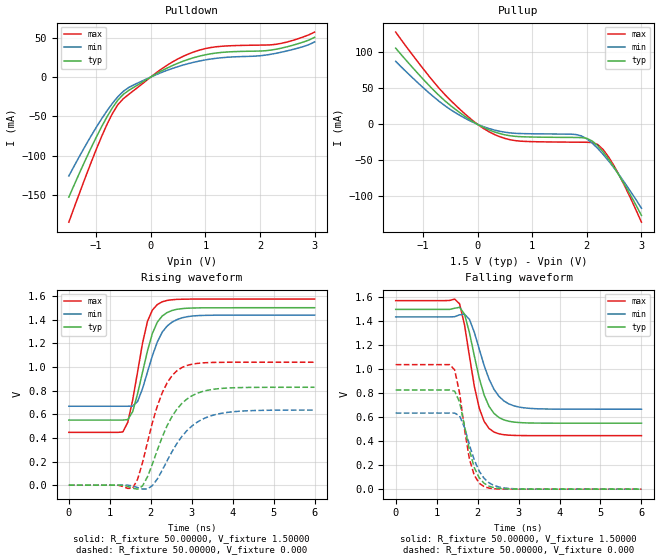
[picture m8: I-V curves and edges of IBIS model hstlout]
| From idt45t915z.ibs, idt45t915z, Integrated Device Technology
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|   Model hstlout
[Model]   hstlout
Model_type   Output
Polarity   Non-Inverting
Vmeas =  0.75000V
C_comp   5.00000pF   5.00000pF   5.00000pF
[Temperature Range]   45.00000   0.14000k   -30.00000
[Voltage Range]   1.50000V   1.40000V   1.60000V
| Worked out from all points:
|   slope of the pulldown table from 0 to 0.225 V, typ, clamps not added: 25.7 ohm
|   slope of the pullup table from 0 to 0.225 V, typ, clamps not added: 27.7 ohm
|   rising waveform, R_fixture 50.00000, V_fixture 1.50000: 20-80 % time 422ps typ, 461ps min, 368ps max; typ from 0.55 V to 1.5 V
|   rising waveform, R_fixture 50.00000, V_fixture 0.000: 20-80 % time 662ps typ, 754ps min, 540ps max; typ from 0 V to 0.828 V
|   falling waveform, R_fixture 50.00000, V_fixture 1.50000: 20-80 % time 419ps typ, 483ps min, 354ps max; typ from 1.5 V to 0.55 V
|   falling waveform, R_fixture 50.00000, V_fixture 0.000: 20-80 % time 340ps typ, 400ps min, 296ps max; typ from 0.828 V to 0 V
[Pulldown]
| voltage   I(typ)   I(min)   I(max)
-1.5V     -152.2mA   -125.4mA   -184mA
-1V       -76.61mA   -64mA      -92.15mA
-700mV    -38.83mA   -33.15mA   -46.03mA
-600mV    -29.09mA   -24.77mA   -34.85mA
-400mV    -16.8mA    -13.12mA   -21.77mA
100mV     4.071mA    3.04mA     5.393mA
500mV     17.6mA     13.29mA    23.07mA
900mV     26.67mA    20.45mA    34.32mA
1.3V      31.24mA    24.53mA    39.05mA
2.3V      35.32mA    30.19mA    41.59mA
2.7V      42.32mA    36.77mA    48.64mA
3V        50.37mA    44.55mA    57.01mA
[Pullup]
| voltage   I(typ)   I(min)   I(max)
-1.5V     106mA      87.68mA    128.3mA
-1V       63.03mA    51.23mA    77.62mA
-600mV    32.8mA     26mA       41.46mA
-100mV    4.501mA    3.42mA     5.936mA
200mV     -7.39mA    -5.559mA   -9.876mA
700mV     -16.74mA   -12.49mA   -22.72mA
1.8V      -18.22mA   -14.08mA   -24.77mA
2V        -19.46mA   -20.18mA   -24.89mA
2.2V      -29.78mA   -33.53mA   -28.11mA
2.3V      -38.45mA   -41.87mA   -35.18mA
2.5V      -59.91mA   -60.81mA   -57.87mA
3V        -126.6mA   -116.6mA   -136mA
[Ramp]
| variable   typ   min   max
dV/dt_r   0.49650/0.71046n   0.38094/0.80872n   0.62340/0.57985n
dV/dt_f   0.56976/0.43675n   0.47046/0.50537n   0.67140/0.37589n
R_load = 50.00000
[Rising Waveform]
R_fixture = 50.00000
V_fixture = 1.50000
C_fixture = 0.000F
R_dut = 6.00000m
L_dut = 3.00000nH
C_dut = 0.20000pF
| time   V(typ)   V(min)   V(max)
0s        550.4mV    667.1mV    446.5mV
1.32ns    550.2mV    667.1mV    450.2mV
1.44ns    554.3mV    667.1mV    531.4mV
1.56ns    622mV      668.4mV    721.8mV
1.68ns    774.8mV    708.2mV    959.6mV
1.92ns    1.135V     956.3mV    1.384V
2.04ns    1.282V     1.093V     1.48V
2.28ns    1.43V      1.293V     1.55V
3ns       1.497V     1.429V     1.573V
6ns       1.5V       1.437V     1.573V
[Rising Waveform]
R_fixture = 50.00000
V_fixture = 0.000
C_fixture = 0.000F
R_dut = 6.00000m
L_dut = 3.00000nH
C_dut = 0.20000pF
| time   V(typ)   V(min)   V(max)
0s        0V         0V         0V
1.56ns    -25.61mV   -6.834mV   -25.24mV
1.8ns     -5.907mV   -32.5mV    190.7mV
2.04ns    178.2mV    -3.565mV   528.3mV
2.28ns    407.3mV    126mV      780.3mV
2.52ns    581.2mV    283.8mV    925.6mV
2.76ns    690.8mV    411.7mV    994.3mV
3.12ns    774.6mV    529.8mV    1.028V
3.72ns    817.6mV    607.2mV    1.038V
6ns       827.5mV    635mV      1.039V
[Falling Waveform]
R_fixture = 50.00000
V_fixture = 1.50000
C_fixture = 0.000F
R_dut = 6.00000m
L_dut = 3.00000nH
C_dut = 0.20000pF
| time   V(typ)   V(min)   V(max)
0s        1.5V       1.437V     1.573V
1.56ns    1.517V     1.454V     1.546V
1.68ns    1.46V      1.46V      1.371V
1.8ns     1.307V     1.417V     1.111V
2.04ns    925.7mV    1.168V     676mV
2.16ns    784.8mV    1.031V     564.9mV
2.4ns     632.1mV    832.9mV    476.3mV
2.64ns    578.1mV    736.5mV    454.2mV
3.12ns    553.8mV    679.2mV    447.1mV
6ns       550.4mV    667.1mV    446.5mV
[Falling Waveform]
R_fixture = 50.00000
V_fixture = 0.000
C_fixture = 0.000F
R_dut = 6.00000m
L_dut = 3.00000nH
C_dut = 0.20000pF
| time   V(typ)   V(min)   V(max)
0s        827.5mV    635.2mV    1.039V
1.32ns    827.6mV    635.2mV    1.039V
1.44ns    817.4mV    634.9mV    995mV
1.56ns    726mV      611.1mV    801mV
1.8ns     325.5mV    369.4mV    250.5mV
1.92ns    178.8mV    242mV      114.4mV
2.16ns    48.59mV    89.58mV    20.38mV
2.4ns     12.37mV    30.67mV    3.691mV
2.76ns    1.798mV    6.18mV     403.3uV
6ns       0V         722.7nV    0V
